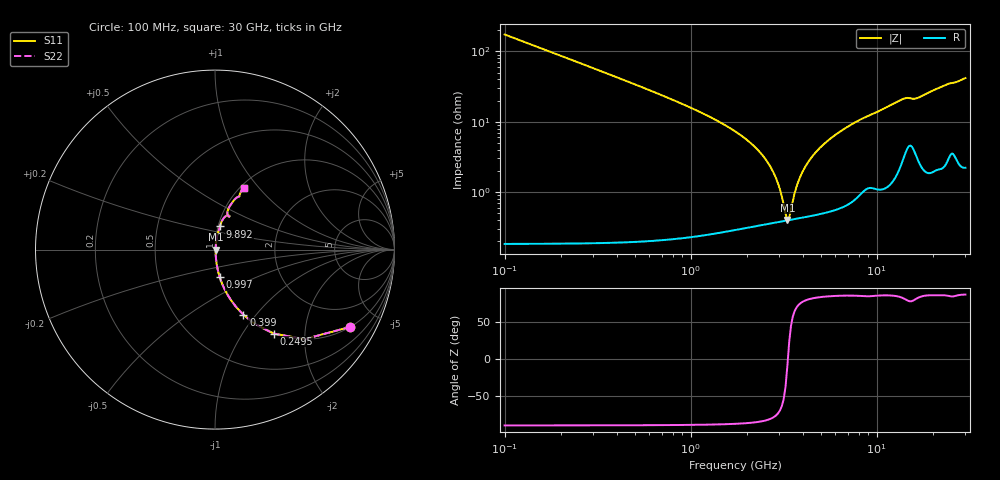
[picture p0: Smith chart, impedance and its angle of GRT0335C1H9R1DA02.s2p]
!Murata Part Number: GRT0335C1H9R1DA02
!These Parameters are Measured in Series Mode Connection
!Data Generated on Jun 19, 2026
!  o--ll--o
!Port1  Port2
!  o------o
!Operation Temp=25[degC], DC Bias Voltage=0[V]
!Freq. Start=100[MHz] Stop=30[GHz] 401[Steps]
# Hz S RI R 50
!Freq.(Hz) S11(Real) S11(Imag) S21(Real) S21(Imag) S12(Real) S12(Imag) S22(Real) S22(Imag)
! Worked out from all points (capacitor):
!   401 points, 100 MHz to 30 GHz, reference 50 ohm
!   read as one part in series: C = 9.1 pF near 249.5 MHz
!   lowest |Z| = 399 mohm at 3.314 GHz (marker M1)
!   series resonance near 3.333 GHz, so ESL is about 250 pH
!   S11 on the Smith chart (normalised r, x): 100 MHz: 1.00, -3.49; 249.5 MHz: 1.00, -1.39; 399 MHz: 1.00, -0.86; 997 MHz: 1.00, -0.32; 9.892 GHz: 1.02, +0.27; 30 GHz: 1.04, +0.84
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1e8  0.753 -0.4307  0.247 0.4307  0.247 0.4307  0.753 -0.4307
2.495e8  0.3273 -0.4679  0.6727 0.4679  0.6727 0.4679  0.3273 -0.4679
3.99e8  0.1582 -0.3628  0.8418 0.3628  0.8418 0.3628  0.1582 -0.3628
6.2325e8  0.0697 -0.251  0.9303 0.251  0.9303 0.251  0.0697 -0.251
9.97e8  0.0268 -0.1545  0.9732 0.1545  0.9732 0.1545  0.0268 -0.1545
2.56675e9  0.00422 -0.0272  0.9958 0.0272  0.9958 0.0272  0.00422 -0.0272
2.86575e9  0.00391 -0.0156  0.9961 0.0156  0.9961 0.0156  0.00391 -0.0156
3.16475e9  0.00387 -0.00533  0.9961 0.00533  0.9961 0.00533  0.00387 -0.00533
3.31425e9  0.00393 -0.000581  0.9961 0.000581  0.9961 0.000581  0.00393 -0.000581
3.46375e9  0.00403 0.00395  0.996 -0.00395  0.996 -0.00395  0.00403 0.00395
3.76275e9  0.00433 0.0125  0.9957 -0.0125  0.9957 -0.0125  0.00433 0.0125
4.06175e9  0.00475 0.0204  0.9952 -0.0204  0.9952 -0.0204  0.00475 0.0204
4.51025e9  0.00557 0.0315  0.9944 -0.0315  0.9944 -0.0315  0.00557 0.0315
5.10825e9  0.00695 0.0451  0.9931 -0.0451  0.9931 -0.0451  0.00695 0.0451
7.1265e9  0.0142 0.0855  0.9858 -0.0855  0.9858 -0.0855  0.0142 0.0855
9.89225e9  0.028 0.1292  0.972 -0.1292  0.972 -0.1292  0.028 0.1292
1.01165e10  0.0289 0.1329  0.9711 -0.1329  0.9711 -0.1329  0.0289 0.1329
1.34055e10  0.0587 0.1856  0.9413 -0.1856  0.9413 -0.1856  0.0587 0.1856
1.505e10  0.0812 0.186  0.9188 -0.186  0.9188 -0.186  0.0812 0.186
2.005825e10  0.0866 0.2488  0.9134 -0.2488  0.9134 -0.2488  0.0866 0.2488
2.50665e10  0.1335 0.295  0.8665 -0.295  0.8665 -0.295  0.1335 0.295
3e10  0.162 0.343  0.838 -0.343  0.838 -0.343  0.162 0.343
